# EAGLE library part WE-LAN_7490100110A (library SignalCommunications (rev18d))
LAN-Transformer WE-LAN 10/100 Base T - Compliant with IEEE 802.3 standards - SMD -- Ethernet -- Power over Ethernet -- 1 Gigabit Ethernet -- Compliant with most IC's for ethernet applications like Intel, AMD, Globespan and Realtek -- Hub, Router, Switch Details see: http://katalog.we-online.de/en/pbs/WE-LAN/S/7490100110A? 2016 (C) Würth Elektronik
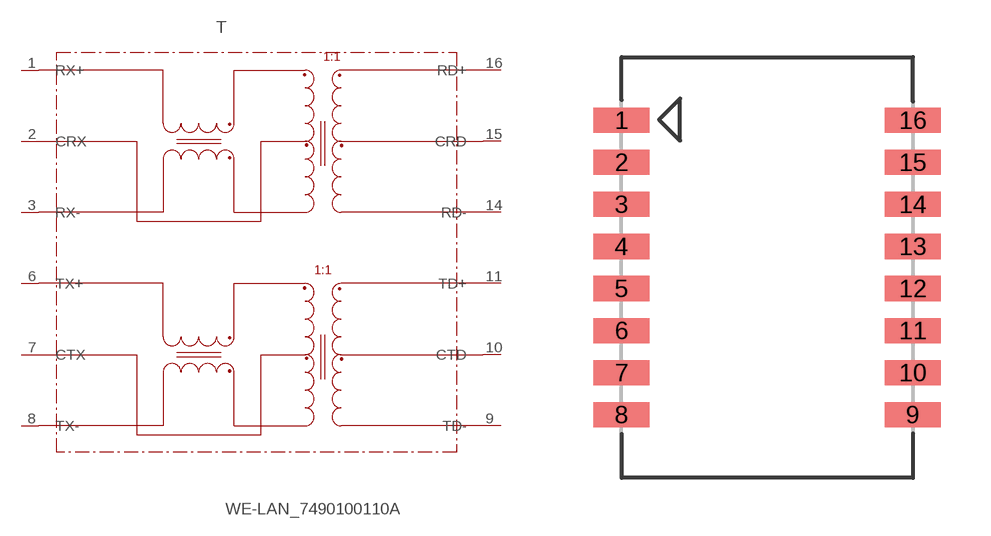
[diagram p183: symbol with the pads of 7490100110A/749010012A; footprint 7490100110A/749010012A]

Designator prefix T

## WE-LAN_7490100110A  [7490100110A/749010012A]
1  RX+
2  CRX
3  RX-
6  TX+
7  CTX
8  TX-
9  TD-
10  CTD
11  TD+
14  RD-
15  CRD
16  RD+

## Footprint 7490100110A/749010012A (pad centres in mm)
smd 1.7 x 0.76: 1 -4.4,4.445; 2 -4.4,3.175; 3 -4.4,1.905; 4 -4.4,0.635; 5 -4.4,-0.635; 6 -4.4,-1.905; 7 -4.4,-3.175; 8 -4.4,-4.445; 9 4.4,-4.445; 10 4.4,-3.175; 11 4.4,-1.905; 12 4.4,-0.635; 13 4.4,0.635; 14 4.4,1.905; 15 4.4,3.175; 16 4.4,4.445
